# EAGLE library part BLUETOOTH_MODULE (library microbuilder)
BLUETOOTH MODULE
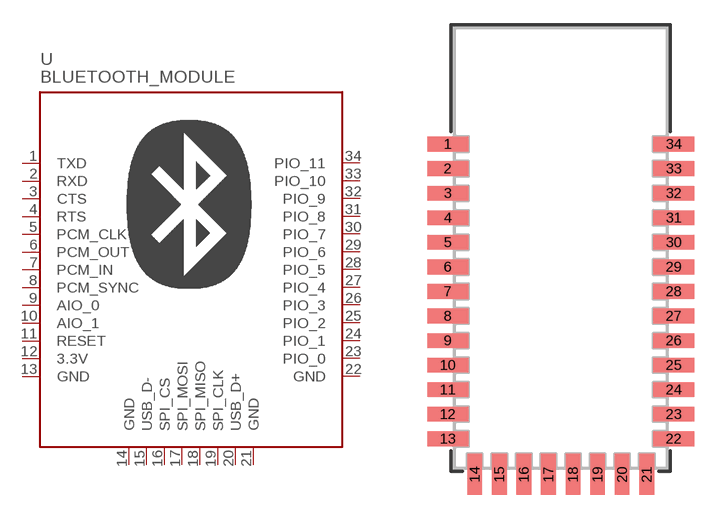
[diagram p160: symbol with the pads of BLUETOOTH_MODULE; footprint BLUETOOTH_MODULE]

Designator prefix U

## BLUETOOTH_MODULE  [BLUETOOTH_MODULE]
1  TXD
2  RXD
3  CTS
4  RTS
5  PCM_CLK
6  PCM_OUT
7  PCM_IN
8  PCM_SYNC
9  AIO_0
10  AIO_1
11  RESET
12  3.3V  pwr
13  GND  pwr
14  GND  pwr
15  USB_D-
16  SPI_CS
17  SPI_MOSI
18  SPI_MISO
19  SPI_CLK
20  USB_D+
21  GND  pwr
22  GND  pwr
23  PIO_0
24  PIO_1
25  PIO_2
26  PIO_3
27  PIO_4
28  PIO_5
29  PIO_6
30  PIO_7
31  PIO_8
32  PIO_9
33  PIO_10
34  PIO_11

## Footprint BLUETOOTH_MODULE (pad centres in mm)
smd 2.5 x 0.9: 1 -6.9,6.35; 2 -6.9,4.85; 3 -6.9,3.35; 4 -6.9,1.85; 5 -6.9,0.35; 6 -6.9,-1.15; 7 -6.9,-2.65; 8 -6.9,-4.15; 9 -6.9,-5.65; 10 -6.9,-7.15; 11 -6.9,-8.65; 12 -6.9,-10.15; 13 -6.9,-11.65; 22 6.9,-11.65; 23 6.9,-10.15; 24 6.9,-8.65; 25 6.9,-7.15; 26 6.9,-5.65; 27 6.9,-4.15; 28 6.9,-2.65; 29 6.9,-1.15; 30 6.9,0.35; 31 6.9,1.85; 32 6.9,3.35; 33 6.9,4.85; 34 6.9,6.35
smd 0.9 x 2.5: 14 -5.25,-13.83; 15 -3.75,-13.83; 16 -2.25,-13.83; 17 -0.75,-13.83; 18 0.75,-13.83; 19 2.25,-13.83; 20 3.75,-13.83; 21 5.25,-13.83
